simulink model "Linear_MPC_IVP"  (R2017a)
settings: Solver=ode4  StartTime=0.0  StopTime=inf  FixedStep=0.1  RelTol=1e-3
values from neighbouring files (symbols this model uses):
  Ac = [0,1,0,0; (m1+m2)*g/(m2*l),0,0,0;0,0,0,1;-m1*g/m2,0,0,0]    [initialization_script.m]
  alpha_op = 0    [initialization_script.m]
  Bc = [0;-1/(m2*l);0;1/m2]    [initialization_script.m]
  F_op = 0    [initialization_script.m]
  v2_op = 0    [initialization_script.m]
  w_op = 0    [initialization_script.m]
  x2_op = 0    [initialization_script.m]
libraries: realtime_pacer_lib x1

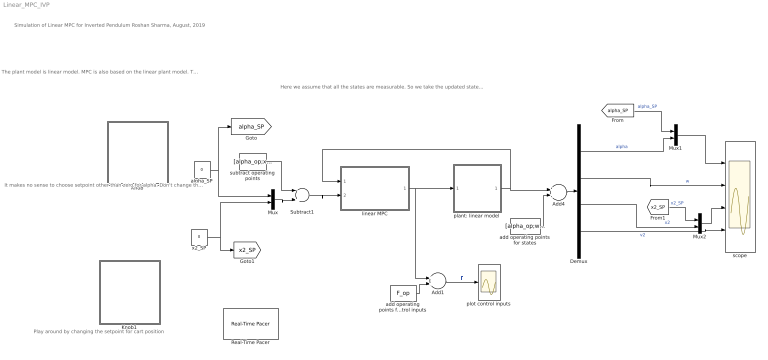
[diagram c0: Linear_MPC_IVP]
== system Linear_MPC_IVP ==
  note: Here we assume that all the states are measurable. So we take the updated states values from the plant model directly back to the linear MPC block. Note: If some of the states are not measurable, then you use the measurements from the plant model and design Kalman filter to estimate the states. You can then take the estimated states back to the MPC block.
  note: It makes no sense to choose setpoint other than zero for alpha. Don't change this knob position
  note: The plant model is linear model. MPC is also based on the linear plant model. Thus there is no plant-model mismatch. Hence controller works perfectly without showing any offsets at the steady state.
  note: Simulation of Linear MPC for Inverted Pendulum Roshan Sharma, August, 2019
  note: Play around by changing the setpoint for cart position
  Add1 : Sum
  Add4 : Sum
  Demux : Demux
  Knob : Subsystem  DialogController=hmiCreateDDGDialog  IsWebBlock=on
  Knob1 : Subsystem  DialogController=hmiCreateDDGDialog  IsWebBlock=on
  Mux : Mux  Inputs=2
  Mux1 : Mux  Inputs=2
  Mux2 : Mux  Inputs=2
  Real-Time Pacer : realtime_pacer_lib/Real-Time Pacer  simTimePerRealTime=1
  Subtract1 : Sum  Inputs=-+
  add operating points for control inputs : Constant  Value=F_op
  add operating points for states : Constant  Value=[alpha_op;w_op;x2_op;v2_op]
  alpha_SP : Constant  Value=0
  linear MPC : Subsystem  TreatAsAtomicUnit=on
  plant: linear model : Subsystem
  plot control inputs : Scope
  scope : Scope  NumInputPorts=4
  subtract operating points : Constant  Value=[alpha_op;x2_op]
  x2_SP : Constant  Value=0
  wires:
  linear MPC/1(delat_u_opt) -> plant: linear model/1(delta_u), Add1/1
  Demux/2 -> scope/2  "w"
  Demux/4 -> scope/4  "v2"
  Demux/1 -> Mux1/2  "alpha"
  Demux/3 -> Mux2/2  "x2"
  plant: linear model/1(delta_x) -> linear MPC/1(delta_x0), Add4/1
  x2_SP/1 -> [x2_SP], Mux/2
  alpha_SP/1 -> Mux/1, [alpha_SP]
  [alpha_SP] -> Mux1/1  "alpha_SP"
  Mux1/1 -> scope/1
  [x2_SP] -> Mux2/1  "x2_SP"
  Mux2/1 -> scope/3
  add operating points for states/1 -> Add4/2
  Mux/1 -> Subtract1/2
  subtract operating points/1 -> Subtract1/1
  Subtract1/1 -> linear MPC/2(delta_r)
  Add1/1 -> plot control inputs/1  "F"
  add operating points for control inputs/1 -> Add1/2
  Add4/1 -> Demux/1

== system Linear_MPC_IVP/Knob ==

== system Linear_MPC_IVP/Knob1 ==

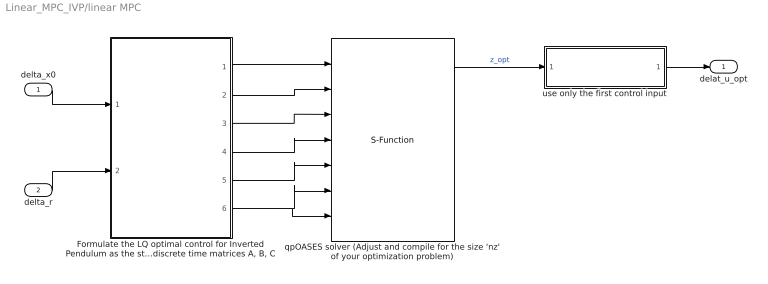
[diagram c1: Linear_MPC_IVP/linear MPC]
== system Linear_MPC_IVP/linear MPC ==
  delta_x0 : Inport
  delta_r : Inport  Port=2
  "Formulate the LQ optimal control for Inverted Pendulum as the standard QP problem. Use MATLAB Function block to construct matrices H, c, Ae, be, zL and zU Use discrete time matrices A, B, C" : ModelReference  ModelNameDialog=Formulate_the_LQ_optimal_con  ModelReferenceVersion=1.93  CopyOfModelProtected=on
  qpOASES solver (Adjust and compile for the size 'nz' of your optimization problem) : S-Function  FunctionName=qpOASES_SQProblem  SFunctionDeploymentMode=off  EnableBusSupport=off
  use only the first control input : MATLAB Function  TreatAsAtomicUnit=on
  delat_u_opt : Outport
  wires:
  qpOASES solver (Adjust and compile for the size 'nz' of your optimization problem)/1 -> use only the first control input/1(z_opt)  "z_opt"
  "Formulate the LQ optimal control for Inverted Pendulum as the standard QP problem. Use MATLAB Function block to construct matrices H, c, Ae, be, zL and zU Use discrete time matrices A, B, C"/1 -> qpOASES solver (Adjust and compile for the size 'nz' of your optimization problem)/1
  "Formulate the LQ optimal control for Inverted Pendulum as the standard QP problem. Use MATLAB Function block to construct matrices H, c, Ae, be, zL and zU Use discrete time matrices A, B, C"/4 -> qpOASES solver (Adjust and compile for the size 'nz' of your optimization problem)/4
  "Formulate the LQ optimal control for Inverted Pendulum as the standard QP problem. Use MATLAB Function block to construct matrices H, c, Ae, be, zL and zU Use discrete time matrices A, B, C"/5 -> qpOASES solver (Adjust and compile for the size 'nz' of your optimization problem)/5
  "Formulate the LQ optimal control for Inverted Pendulum as the standard QP problem. Use MATLAB Function block to construct matrices H, c, Ae, be, zL and zU Use discrete time matrices A, B, C"/2 -> qpOASES solver (Adjust and compile for the size 'nz' of your optimization problem)/2
  "Formulate the LQ optimal control for Inverted Pendulum as the standard QP problem. Use MATLAB Function block to construct matrices H, c, Ae, be, zL and zU Use discrete time matrices A, B, C"/6 -> qpOASES solver (Adjust and compile for the size 'nz' of your optimization problem)/7, qpOASES solver (Adjust and compile for the size 'nz' of your optimization problem)/6
  "Formulate the LQ optimal control for Inverted Pendulum as the standard QP problem. Use MATLAB Function block to construct matrices H, c, Ae, be, zL and zU Use discrete time matrices A, B, C"/3 -> qpOASES solver (Adjust and compile for the size 'nz' of your optimization problem)/3
  use only the first control input/1(delta_u_opt) -> delat_u_opt/1
  delta_x0/1 -> "Formulate the LQ optimal control for Inverted Pendulum as the standard QP problem. Use MATLAB Function block to construct matrices H, c, Ae, be, zL and zU Use discrete time matrices A, B, C"/1
  delta_r/1 -> "Formulate the LQ optimal control for Inverted Pendulum as the standard QP problem. Use MATLAB Function block to construct matrices H, c, Ae, be, zL and zU Use discrete time matrices A, B, C"/2

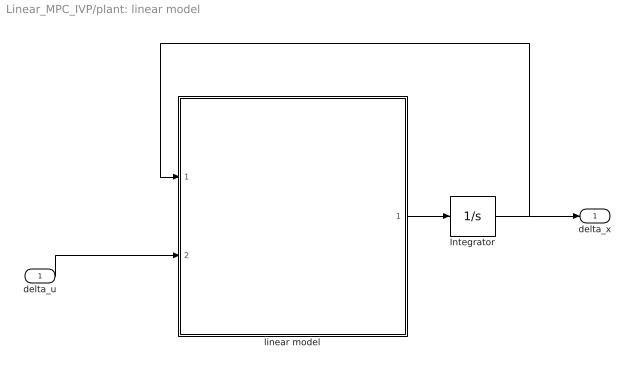
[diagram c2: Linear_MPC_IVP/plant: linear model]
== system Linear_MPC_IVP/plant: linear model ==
  delta_u : Inport  OutDataTypeStr=double  PortDimensions=1  SampleTime=[0.10000000000000001,0]
  Integrator : Integrator  InitialCondition=[0,0,0,0]  ContinuousStateAttributes='model_integrator'
  linear model : MATLAB Function  TreatAsAtomicUnit=on  SystemSampleTime=0.1
  delta_x : Outport  OutDataTypeStr=double  PortDimensions=4  SampleTime=0
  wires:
  linear model/1(delta_x_dot) -> Integrator/1
  Integrator/1 -> delta_x/1, linear model/1(delta_x)
  delta_u/1 -> linear model/2(delta_u)

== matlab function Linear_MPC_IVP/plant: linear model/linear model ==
function delta_x_dot = linear_model(delta_x,delta_u,Ac, Bc)

%linear state space model equation
delta_x_dot = Ac*delta_x + Bc*delta_u;

== matlab function Linear_MPC_IVP/linear MPC/use only the first 
control input ==
function delta_u_opt = select_first(z_opt)

delta_u_opt = z_opt(1);
